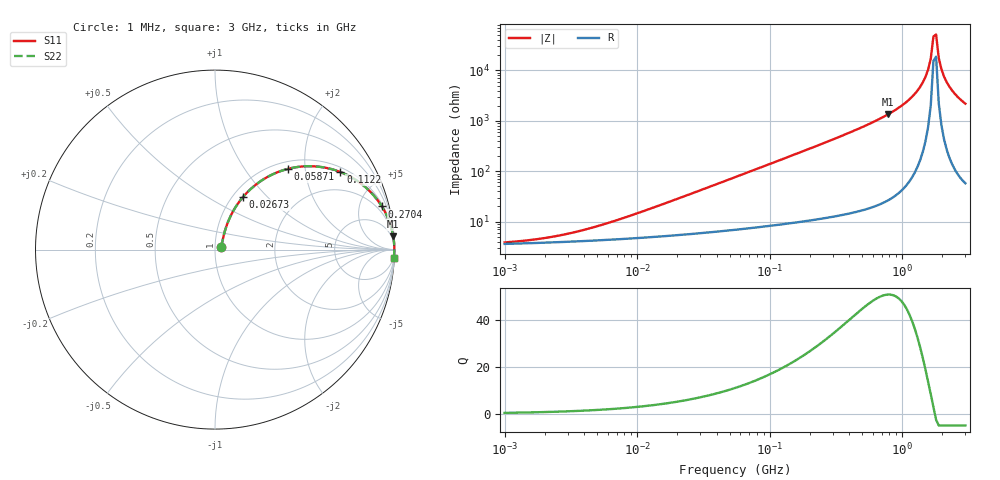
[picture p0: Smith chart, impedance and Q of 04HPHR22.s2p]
# MHz S MA R 50
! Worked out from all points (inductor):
!   174 points, 1 MHz to 3 GHz, reference 50 ohm
!   read as one part in series: L = 220 nH near 10.59 MHz
!   highest Q = 50.9 at 783.9 MHz (marker M1), where L = 274 nH
!   self-resonance near 1.722 GHz
!   S11 on the Smith chart (normalised r, x): 1 MHz: 1.07, +0.03; 26.73 MHz: 1.11, +0.74; 58.71 MHz: 1.14, +1.62; 112.2 MHz: 1.17, +3.12; 270.4 MHz: 1.24, +7.65; 3 GHz: 2, -44
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1  0.03731 20.2  0.9651 -0.8  0.9651 -0.8  0.03731 20.2
3.8271  0.0642 49.3  0.9594 -2.9  0.9594 -2.9  0.0642 49.3
14.6467  0.1951 65.1  0.9347 -10.9  0.9347 -10.9  0.1951 65.1
26.7317  0.3339 61.9  0.8928 -19.3  0.8928 -19.3  0.3339 61.9
56.0545  0.5895 48.9  0.757 -36.0  0.757 -36.0  0.5895 48.9
58.7096  0.6069 47.9  0.7443 -37.2  0.7443 -37.2  0.6069 47.9
112.226  0.8217 31.7  0.5267 -55.1  0.5267 -55.1  0.8217 31.7
214.526  0.939 18.2  0.3118 -69.8  0.3118 -69.8  0.939 18.2
270.38  0.9603 14.5  0.2508 -73.7  0.2508 -73.7  0.9603 14.5
783.883  0.9958 4.2  0.07375 -84.6  0.07375 -84.6  0.9958 4.2
821.013  0.9963 3.9  0.06876 -84.9  0.06876 -84.9  0.9963 3.9
1135.12  0.9984 2.1  0.03729 -86.5  0.03729 -86.5  0.9984 2.1
1430.66  0.9991 1.0  0.0173 -86.6  0.0173 -86.6  0.9991 1.0
1569.41  0.9993 0.6  0.009626 -85.3  0.009626 -85.3  0.9993 0.6
1643.75  0.9993 0.3  0.005833 -82.8  0.005833 -82.8  0.9993 0.3
1721.61  0.9993 0.1  0.002112 -70.7  0.002112 -70.7  0.9993 0.1
1803.15  0.9993 -0.1  0.001929 68.6  0.001929 68.6  0.9993 -0.1
1888.56  0.9993 -0.3  0.005639 82.4  0.005639 82.4  0.9993 -0.3
1978.02  0.9992 -0.5  0.00943 85.0  0.00943 85.0  0.9992 -0.5
2071.71  0.9992 -0.8  0.01325 86.0  0.01325 86.0  0.9992 -0.8
2380.27  0.9988 -1.4  0.02492 86.6  0.02492 86.6  0.9988 -1.4
3000  0.9978 -2.6  0.04553 85.9  0.04553 85.9  0.9978 -2.6
